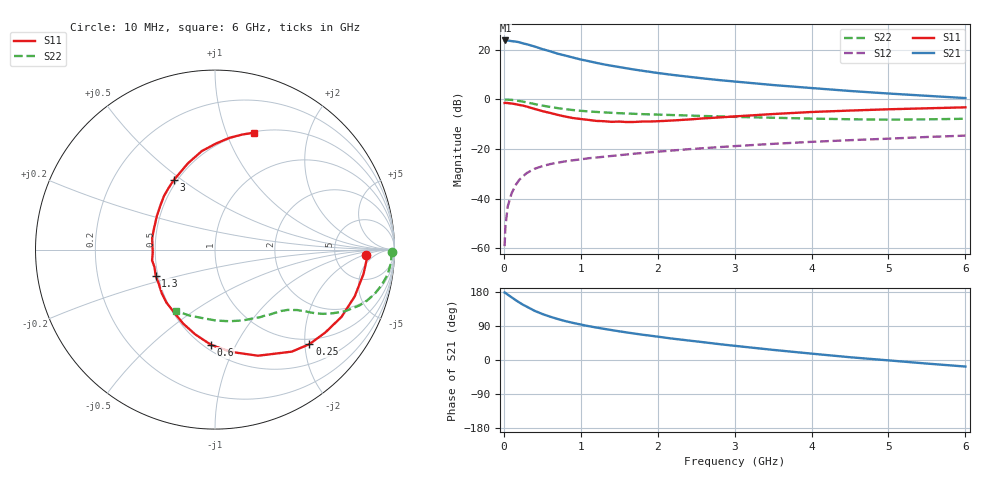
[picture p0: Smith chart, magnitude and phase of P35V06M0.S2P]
! SIEMENS Small Signal Semiconductors
! BFP181
! Si NPN RF Bipolar Junction Transistor in SOT143
! VCE = 5 V  IC = 6 mA
! Common Emitter S-Parameters:  March  1996
# GHz  S  MA  R  50
!  f  S11  S21  S12  S22
! GHz  MAG  ANG  MAG  ANG  MAG  ANG  MAG  ANG
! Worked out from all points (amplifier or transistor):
!   36 points, 10 MHz to 6 GHz, reference 50 ohm
!   highest |S21| = 23.7 dB at 20 MHz (marker M1)
!   |S21| within 3 dB of that: start of sweep to 454.7 MHz
!   unconditionally stable (mu >= 1): 1.608 GHz to end of sweep
!   at 250 MHz: K = 0.24, MSG = 26.7 dB, |S12| = -31.0 dB
!   at 1.4 GHz: K = 0.94, MSG = 18.2 dB, |S12| = -22.8 dB
!   at 6 GHz: K = 1.04, MAG = 6.3 dB, |S12| = -14.6 dB
!   S11 on the Smith chart (normalised r, x): 10 MHz: 11, -2; 250 MHz: 0.89, -2.10; 600 MHz: 0.54, -0.80; 1.3 GHz: 0.49, -0.16; 3 GHz: 0.48, +0.47; 6 GHz: 0.51, +1.26
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0.01  0.8411 -2.1  15.24 178.1  0.0011 77.2  0.9888 -0.7
0.02  0.8467 -3.8  15.28 177.2  0.0027 95.3  0.9837 -1.6
0.05  0.8386 -9.3  15.25 172.5  0.0069 87.3  0.9834 -4.2
0.15  0.7983 -28.0  14.51 158.5  0.0184 75.1  0.95 -11.9
0.2  0.7688 -36.9  14.09 151.9  0.0238 70.5  0.9239 -15.4
0.25  0.7445 -45.1  13.32 145.8  0.0282 66.7  0.8938 -18.5
0.3  0.7111 -53.1  12.79 140.5  0.0328 63.4  0.8634 -21.1
0.4  0.6381 -67.9  11.55 129.8  0.0398 58.0  0.8011 -25.4
0.5  0.5769 -81.1  10.25 121.4  0.0449 53.0  0.7457 -28.4
0.6  0.5311 -92.4  9.261 114.4  0.0494 50.1  0.7012 -30.7
0.7  0.4843 -103.3  8.273 108.2  0.0528 48.1  0.6626 -32.4
0.8  0.4488 -113.3  7.581 102.6  0.0562 46.4  0.6326 -33.5
0.9  0.4182 -122.8  6.912 97.9  0.0591 45.2  0.606 -34.5
1.1  0.3839 -140.5  5.865 89.4  0.0649 43.5  0.5687 -36.3
1.3  0.3614 -156.1  5.038 82.3  0.0696 42.5  0.5441 -38.2
1.7  0.3494 175.8  3.953 69.7  0.0803 41.6  0.509 -42.0
2.2  0.3741 149.9  3.086 56.2  0.0931 39.8  0.4802 -47.9
3  0.4511 120.5  2.276 37.4  0.1139 35.7  0.4416 -59.6
3.5  0.504 107.4  1.934 26.7  0.1265 32.8  0.4244 -68.4
4.5  0.5919 89.3  1.468 7.3  0.1499 25.9  0.3956 -89.1
5.5  0.6575 76.9  1.173 -9.4  0.1738 19.9  0.394 -111.0
6  0.6878 71.4  1.057 -17.3  0.1853 16.2  0.405 -122.2
